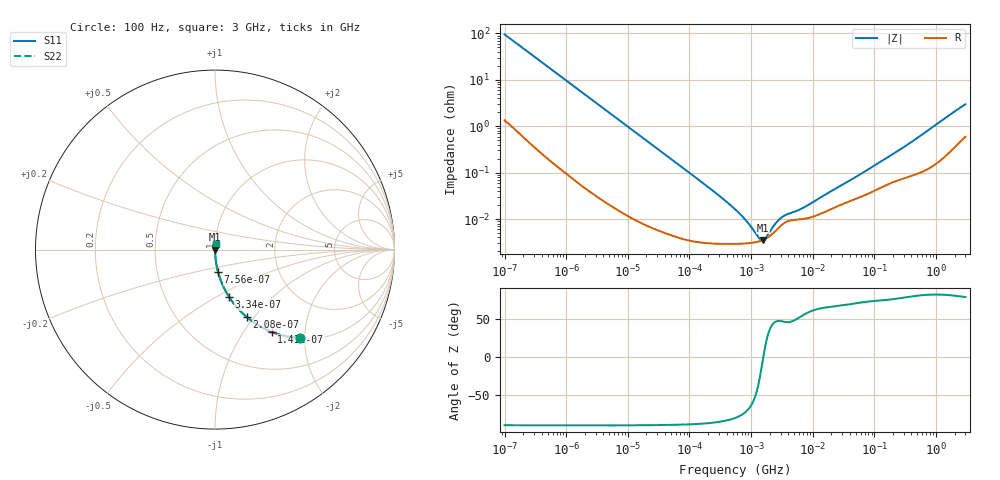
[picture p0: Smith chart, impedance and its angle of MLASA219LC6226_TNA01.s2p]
! MLASA219LC6226_TNA01  S-PARAMETER MODEL  ( Standard Model )
! Model Generated by TAIYO YUDEN Corporation (http://www.ty-top.com)
! Version 1.0
! TAIYO YUDEN Control No. 220601
! Copyright(c) 2014 TAIYO YUDEN CO.,LTD. All Rights Reserved.
! Product Description (link to TY-COMPAS)
! https://ds.yuden.co.jp/TYCOMPAS/or/detail?pn=MLASA219LC6226MTNA01&u=M
! Products Name : Multilayer Ceramic Capacitors
! Characteristics :
!  Capacitance : 22 [uF] , Rated Voltage : 4 [V] , TCC : X6S
!  Case Size : 2.0 x 1.25 / 0.079 x 0.049 [mm/inch] , Thickness : 0.85 / 0.033 [mm/inch]
!  (Conditions: Temperature = 25 [degC] , DC Bias Voltage = 0 [V])
! External Node Assignments :
!  1  o---| |---o  2
! GND o---------o GND
! Frequency Range : 100Hz  -  3GHz  [ 401 STEP ]
# MHZ S RI R 50
! Freq[MHz].  S11 Real  S11 Imag  S21 Real  S21 Imag  S12 Real  S12 Imag  S22 Real  S22 Imag
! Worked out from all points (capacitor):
!   401 points, 100 Hz to 3 GHz, reference 50 ohm
!   read as one part in series: C = 16.7 uF near 109 Hz
!   lowest |Z| = 3.52 mohm at 1.539 MHz (marker M1)
!   series resonance near 1.577 MHz, so ESL is about 610 pH
!   S11 on the Smith chart (normalised r, x): 100 Hz: 1.03, -1.90; 141 Hz: 1.02, -1.35; 208 Hz: 1.01, -0.92; 334 Hz: 1.01, -0.58; 756 Hz: 1.00, -0.26; 3 GHz: 1.01, +0.06
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0.0001  0.4748 -0.4924  0.5252 0.4924  0.5252 0.4924  0.4748 -0.4924
0.000141  0.3159 -0.4583  0.6841 0.4583  0.6841 0.4583  0.3159 -0.4583
0.000208  0.1778 -0.3764  0.8222 0.3764  0.8222 0.3764  0.1778 -0.3764
0.000334  0.0789 -0.2641  0.9211 0.2641  0.9211 0.2641  0.0789 -0.2641
0.000756  0.0172 -0.1252  0.9828 0.1252  0.9828 0.1252  0.0172 -0.1252
0.001788  0.00344 -0.054  0.9966 0.054  0.9966 0.054  0.00344 -0.054
0.005476  0.000504 -0.0178  0.9995 0.0178  0.9995 0.0178  0.000504 -0.0178
0.031977  6.53e-05 -0.00308  0.9999 0.00308  0.9999 0.00308  6.53e-05 -0.00308
0.221826  3e-05 -0.00044  1 0.00044  1 0.00044  3e-05 -0.00044
0.547723  2.92e-05 -0.000161  1 0.000161  1 0.000161  2.92e-05 -0.000161
0.740304  2.95e-05 -0.000106  1 0.000106  1 0.000106  2.95e-05 -0.000106
0.806856  2.98e-05 -9.21e-05  1 9.21e-05  1 9.21e-05  2.98e-05 -9.21e-05
1.53882  3.51e-05 -3.19e-06  1 3.19e-06  1 3.19e-06  3.51e-05 -3.19e-06
2.81117  6.51e-05 7.05e-05  0.9999 -7.05e-05  0.9999 -7.05e-05  6.51e-05 7.05e-05
3.79959  8.79e-05 9e-05  0.9999 -9e-05  0.9999 -9e-05  8.79e-05 9e-05
6.368694  9.87e-05 0.000131  0.9999 -0.000131  0.9999 -0.000131  9.87e-05 0.000131
9.794414  0.000111 0.000197  0.9999 -0.000197  0.9999 -0.000197  0.000111 0.000197
50.26955  0.000272 0.000763  0.9997 -0.000763  0.9997 -0.000763  0.000272 0.000763
175.1444  0.000581 0.00218  0.9994 -0.00218  0.9994 -0.00218  0.000581 0.00218
380.0727  0.00085 0.00428  0.9991 -0.00428  0.9991 -0.00428  0.00085 0.00428
1868.531  0.00355 0.0191  0.9964 -0.0191  0.9964 -0.0191  0.00355 0.0191
3000  0.00672 0.0288  0.9933 -0.0288  0.9933 -0.0288  0.00672 0.0288
